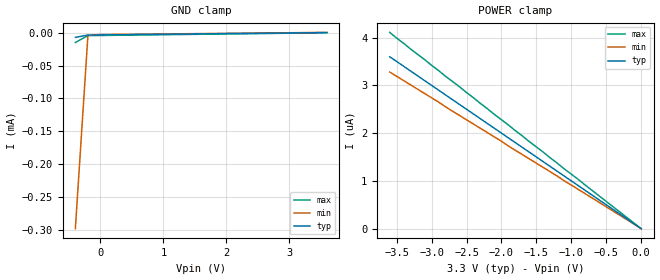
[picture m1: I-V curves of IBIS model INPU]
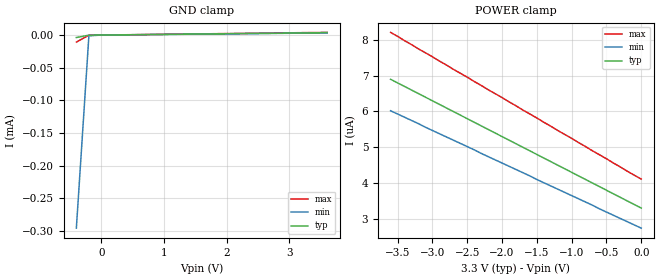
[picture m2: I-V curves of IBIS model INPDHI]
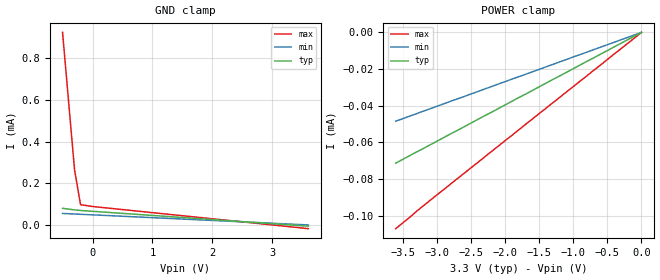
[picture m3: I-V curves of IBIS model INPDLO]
|   Texas Instruments Incorporated
|   Data Transmissions Products
|   IBIS Model for ISO723x4x
|   16DW SOIC Package
[IBIS Ver]   3.2
[Comment char]   |_char
[File name]   iso1176_3.ibs
[File Rev]   1.0
[Date]   11July08
[Source]   File originated at Texas Instruments Incorporated.
   Data Transmission Products Group.
[Notes]
[Disclaimer]
(C) Copyright Texas Instruments Incorporated 2002
   All rights reserved
  Texas Instruments Incorporated hereby grants the user of this IBIS
model a non-exclusive, nontransferable license to use this IBIS model
under the following terms.  Before using this IBIS model, the user
should read this license.  If the user does not accept these terms,
the IBIS model should be returned to Texas Instruments within 30 days.
  The user is granted this license only to use the IBIS model and
is not granted rights to sell, load, rent, lease or license the IBIS
model in whole or in part, or in modified form to anyone other than
user.  User may modify the IBIS model to suit its specific applications
but rights to derivative works and such modifications shall belong to
Texas Instruments.
  This IBIS model is provided on an "AS IS" basis and Texas Instruments
makes absolutely no warranty with respect to the information contained
herein.  TEXAS INSTRUMENTS DISCLAIMS AND CUSTOMER WAIVES ALL WARRANTIES,
EXPRESS OR IMPLIED, INCLUDING WARRANTIES OF MERCHANTABILITY OR FITNESS
FOR A PARTICULAR PURPOSE. The entire risk as to quality and performance
is with the Customer. ACCORDINGLY, IN NO EVENT SHALL THE COMPANY BE LIABLE
FOR ANY DAMAGES, WHETHER IN CONTRACT OR TORT,INCLUDING ANY LOST PROFITS
OR OTHER INCIDENTAL, CONSEQUENTIAL, EXEMPLARY, OR PUNITIVE DAMAGES ARISING
OUT OF THE USE OR APPLICATION OF THE IBIS model provided in this package.
Further, Texas Instruments reserves the right to discontinue or make changes
without notice to any product herein to improve reliability, function, or
design. Texas Instruments does not convey any license under patent rights
or any other intellectual property rights, including those of third parties.
Contact Texas Instruments at ATTN:DATA TRANSMISSIONS
[Copyright]   Copyright 2002, Texas Instruments, All Rights Reserved
[Component]   ISO1176DW
[Manufacturer]  Texas Instruments Incorporated
[Package]
|   typ   min   max
R_pkg   0.04817   0.03432   0.09530
L_pkg   2.4595nH   1.6904nH   4.7034nH
C_pkg   0.847pF   0.428pF   1.397pF
[Pin]   signal_name   model_name   R_pin   L_pin   C_pin
1   VCC1   POWER   0.03455  3.39778n  0.89677p
2   GND1   GND   0.03432  3.12613n  0.84706p
3   R   OUTR   0.04265  1.85523n  0.57831p
4   REB   INPU   0.03948  1.69049n  0.59300p
5   DE   INPDHI   0.03943  1.70546n  0.55709p
6   D   INPU   0.04257  1.86953n  0.56379p
7   PV   INPDLO   0.04783  1.99000n  0.60148p
8   GND1   GND   0.03740  4.70338n  1.39696p
9   GND2   GND   0.03763  4.61305n  1.39587p
10   ISODE   OUTDE   0.08703  5.01514n  1.58483p
11   NC   NC   0.07132  2.45946n  0.43321p
12   A   DRVR/REC_BI   0.06147  2.13194n  0.42769p
13   B   DRVR/REC_BI   0.07288  2.39260n  0.48001p
14   NC   NC   0.09530  3.03704n  0.47622p
15   GND2   GND   0.04817  4.23145n  0.93567p
16   VCC2   POWER   0.04790  4.51154n  0.99405p
[Diff_pin]   inv_pin   vdiff   tdelay_typ   tdelay_min   tdelay_max
| The 'A' pin is Diff_pin and the 'B' pin is the inv_pin
12   13   0.200   0 0 0
| Models and submodels in the file (6): INPU (Input), INPDHI (Input), INPDLO (Input), OUTDE (3-state), OUTR (3-state), DRVR/REC_BI (I/O)
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|   Driver Input / Receiver Enable Model
[Model]   INPU
Model_type   Input
|Signals   REB,D
Vinh = 2.0
Vinl = 0.8
|   typ   min   max
C_comp   1.3pF   1.1pF   1.5pF
|   typ   min   max
[Temperature Range]   27   -40   125
[Voltage range]   3.3V   3.0V   3.6V
[GND_clamp]
|   Voltage   I(typ)   I(min)   I(max)
-400mV    -7.04uA    -298uA     -14.8uA
-200mV    -3.5uA     -3.91uA    -4.34uA
0V        -3.3uA     -2.74uA    -4.11uA
3.6V      300nA      549nA      14.4pA
[Power_clamp]
| Note that the[POWER_clamp]voltage table is referenced to Vcc
| and is calculated using Vtable=Vcc - Vmeasured.
|   Voltage   I(typ)   I(min)   I(max)
-3.6V     3.6uA      3.28uA     4.11uA
-2.9V     2.9uA      2.65uA     3.31uA
-2.8V     2.8uA      2.55uA     3.19uA
0V        0A         0A         0A
|   Driver Enable
[Model]   INPDHI
Model_type   Input
|Signals   DE
Vinh = 2.0
Vinl = 0.8
|   typ   min   max
C_comp   1.3pF   1.1pF   1.5pF
|   typ   min   max
[Temperature Range]   27   -40   125
[Voltage range]   3.3V   3.0V   3.6V
[GND_clamp]
|   Voltage   I(typ)   I(min)   I(max)
-400mV    -3.79uA    -296uA     -10.8uA
-200mV    -202nA     -1.2uA     -230nA
0V        0A         0A         0A
3.6V      3.6uA      3.28uA     4.11uA
[Power_clamp]
| Note that the[POWER_clamp]voltage table is referenced to Vcc
| and is calculated using Vtable=Vcc - Vmeasured.
|   Voltage   I(typ)   I(min)   I(max)
-3.6V     6.9uA      6.02uA     8.21uA
-500mV    3.8uA      3.19uA     4.68uA
-200mV    3.5uA      2.92uA     4.33uA
0V        3.3uA      2.74uA     4.11uA
|   PV Enable Model
[Model]   INPDLO
Model_type   Input
|Signals   PV
Vinh = 2.0
Vinl = 0.8
|   typ   min   max
C_comp   1.3pF   1.1pF   1.5pF
|   typ   min   max
[Temperature Range]   27   -40   125
[Voltage range]   3.3V   3.6V   3.0V
[GND_clamp]
|   Voltage   I(typ)   I(min)   I(max)
-500mV    79.7uA     55.1uA     923uA
-300mV    72.2uA     52.4uA     264uA
-200mV    69.3uA     51.1uA     97uA
3.6V      -5.94uA    -12.9pA    -17.8uA
[Power_clamp]
| Note that the[POWER_clamp]voltage table is referenced to Vcc
| and is calculated using Vtable=Vcc - Vmeasured.
|   Voltage   I(typ)   I(min)   I(max)
-3.6V     -71.3uA    -48.4uA    -107uA
-3.3V     -65.3uA    -44.4uA    -97.7uA
-3V       -59.4uA    -40.3uA    -88.7uA
0V        0A         0A         0A
